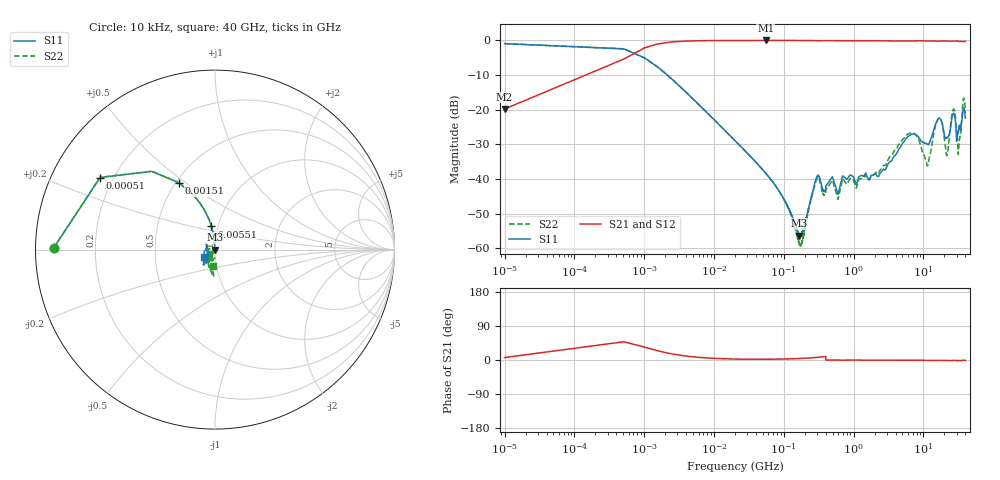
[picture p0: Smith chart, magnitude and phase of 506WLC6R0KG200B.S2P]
!  American Technical Ceramics  Date:  3/15/2011
!  One Norden Lane
!  Huntington Station,  NY.  11746-2102
!  Tel:  (631) 622-4700  Fax:  (631) 622-4748
!  Part Number  506WLC6R0KT200B
!  Description:  Ultra-Broadband Inductor
!  Application:  Ultra-broadband DC block decoupling, bias tee
# GHZ S DB R 50
! Freq  |S11|  S11 Ph  |S21|  S21 Ph  |S12|  S12 Ph  |S22|  S22 Ph
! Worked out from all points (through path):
!   1201 points, 10 kHz to 40 GHz, reference 50 ohm
!   highest |S21| = -0.01 dB at 55.01 MHz (marker M1); lowest = -19.8 dB at 10 kHz (marker M2)
!   lowest |S11| = -56.3 dB at 167.5 MHz (marker M3), VSWR 1.00, Z = 49.9 + j0.0472 ohm
!   |S11| at or under -10 dB: 2.16 MHz to end of sweep
!   |S22| runs from -59.3 to -0.9 dB; largest |S21 - S12| = 0.0041
!   S11 on the Smith chart (normalised r, x): 10 kHz: 0.05, +0.00; 510 kHz: 0.15, +0.28; 1.51 MHz: 0.52, +0.47; 5.51 MHz: 0.93, +0.24; 40 GHz: 0.88, -0.07
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1e-05  -0.93 179.4  -19.78 6.5  -19.76 6.3  -0.92 179.4
0.00051  -2.43 147.9  -5.38 48.2  -5.36 48.1  -2.42 147.8
0.00151  -7.46 118.5  -1.10 25.1  -1.10 25.0  -7.45 118.3
0.00201  -9.49 112.3  -0.66 19.6  -0.66 19.6  -9.48 112.0
0.00551  -17.69 99.0  -0.10 7.6  -0.10 7.6  -17.69 98.5
0.02001  -28.87 94.6  -0.02 2.5  -0.02 2.5  -28.88 93.0
0.05501  -38.27 97.3  -0.01 2.0  -0.01 2.0  -38.33 93.2
0.11101  -47.38 109.2  -0.01 2.8  -0.01 2.8  -47.58 99.7
0.16751  -56.26 162.1  -0.02 3.9  -0.01 3.9  -58.64 150.2
0.252  -44.60 -125.2  -0.03 5.6  -0.03 5.6  -45.02 -129.9
0.3075  -38.95 -155.1  -0.09 7.0  -0.09 7.0  -39.54 -164.2
0.378  -43.53 -165.7  -0.06 8.8  -0.06 8.8  -44.63 -173.7
3.271  -35.07 -131.2  -0.13 -0.6  -0.13 -0.6  -33.65 -145.0
7.033  -27.00 -117.7  -0.15 -0.7  -0.16 -0.7  -26.62 -121.3
11.488  -29.91 -159.4  -0.13 -0.9  -0.13 -1.0  -36.13 -127.9
16.834  -22.39 -118.0  -0.19 -1.0  -0.19 -1.0  -22.41 -110.3
21.784  -28.10 -177.7  -0.18 -1.4  -0.18 -1.5  -33.11 -138.3
27.13  -20.98 -122.3  -0.24 -1.0  -0.24 -1.0  -19.80 -108.0
30.1  -28.72 -134.6  -0.08 -1.3  -0.08 -1.4  -26.04 -93.8
31.684  -26.67 153.5  -0.24 -1.7  -0.25 -1.8  -32.73 -176.1
37.327  -19.78 -125.9  -0.34 -0.7  -0.34 -0.8  -16.86 -96.7
40  -22.41 -146.7  -0.29 -1.3  -0.29 -1.3  -20.94 -96.3
